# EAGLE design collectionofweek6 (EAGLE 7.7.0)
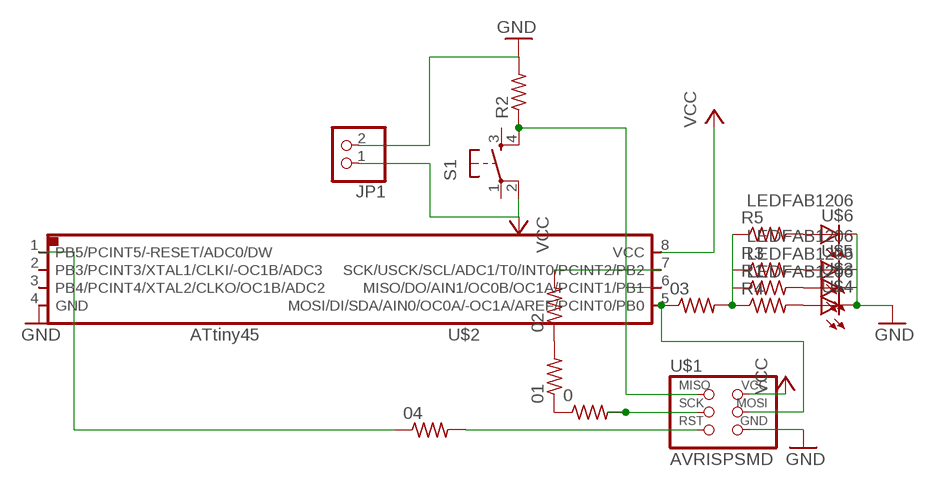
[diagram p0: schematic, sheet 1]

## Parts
0  RES-US1206FAB  [R1206FAB]
01  RES-US1206FAB  [R1206FAB]
02  RES-US1206FAB  [R1206FAB]
03  RES-US1206FAB  [R1206FAB]
04  RES-US1206FAB  [R1206FAB]
JP1  PINHD-1X2  [1X02]
R1  RES-US1206FAB  [R1206FAB]
R2  RES-US1206FAB  [R1206FAB]
R3  RES-US1206FAB  [R1206FAB]
R4  RES-US1206FAB  [R1206FAB]
R5  RES-US1206FAB  [R1206FAB]
S1  6MM_SWITCH6MM_SWITCH  [6MM_SWITCH]
U$1  AVRISPSMD  [2X03SMD]
U$2  ATTINY45SI  [SOIC8]
U$3  LEDFAB1206  [LED1206FAB]
U$4  LEDFAB1206  [LED1206FAB]
U$5  LEDFAB1206  [LED1206FAB]
U$6  LEDFAB1206  [LED1206FAB]

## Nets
GND: JP1.2 R2.2 U$1.6(GND) U$2.4(GND) U$3.2(C) U$4.2(C) U$5.2(C) U$6.2(C)
N$1: 03.1 U$1.4(MOSI) U$2.5(MOSI/DI/SDA/AIN0/OC0A/-OC1A/AREF/PCINT0/PB0)
N$2: R4.2 U$4.1(A)
N$3: R2.1 S1.4(S1) U$1.1(MISO) U$2.6(MISO/DO/AIN1/OC0B/OC1A/PCINT1/PB1)
N$4: 04.1 U$2.1(PB5/PCINT5/-RESET/ADC0/DW)
N$5: 03.2 R1.1 R3.1 R4.1 R5.1
N$6: 0.2 U$1.3(SCK)
N$7: R1.2 U$3.1(A)
N$8: R3.2 U$5.1(A)
N$9: R5.2 U$6.1(A)
N$10: 04.2 U$1.5(RST)
N$11: 0.1 01.1
N$12: 02.2 U$2.7(SCK/USCK/SCL/ADC1/T0/INT0/PCINT2/PB2)
N$13: 01.2 02.1
VCC: JP1.1 S1.2(P1) U$1.2(VCC) U$2.8(VCC)
Unconnected: S1.1(P) S1.3(S) U$2.2(PB3/PCINT3/XTAL1/CLKI/-OC1B/ADC3) U$2.3(PB4/PCINT4/XTAL2/CLKO/OC1B/ADC2)

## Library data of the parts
0 01-04 R1-R5 = fab:RES-US: Resistor (US Symbol)
JP1 = pinhead:PINHD-1X2: PIN HEADER
S1 = fab:6MM_SWITCH: OMRON SWITCH
U$1 = fab:AVRISP
U$2 = fab:ATTINY45
U$3-U$6 = fab:LED: LED

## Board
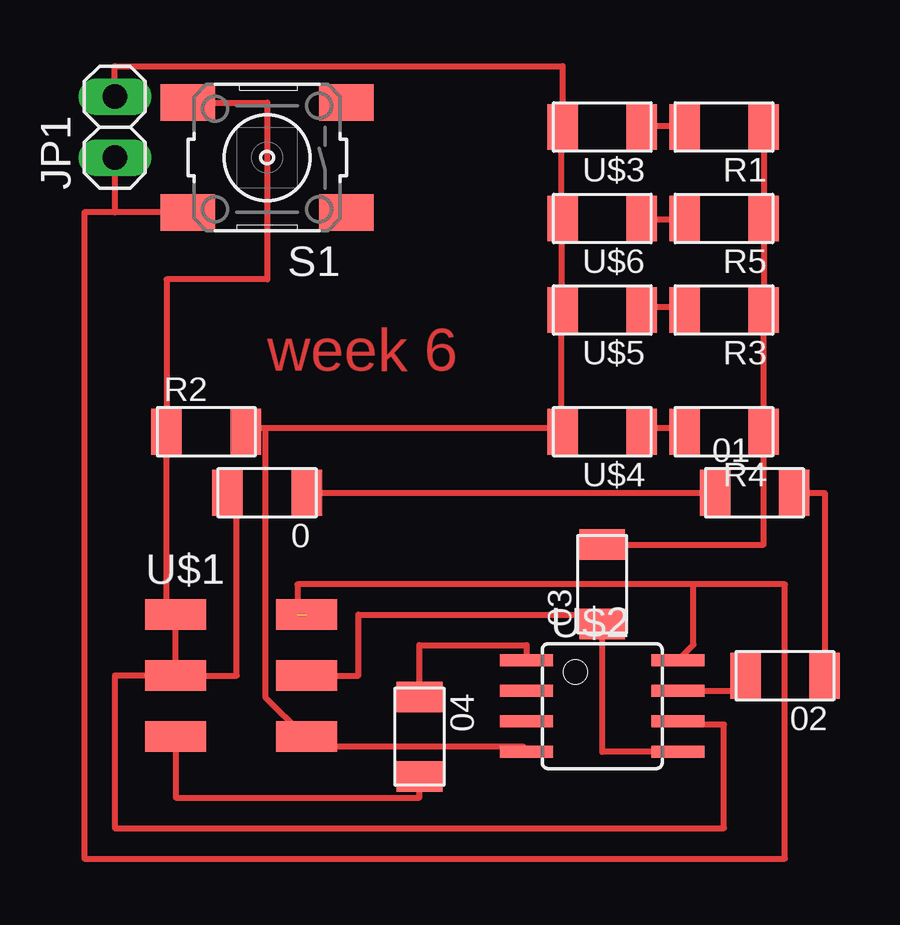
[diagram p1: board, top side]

No outline drawn. Coordinates in mm, seen from the top.
Copper layers (1*16): Top 0.035mm / dielectric 1.5mm / Bottom 0.035mm
Design rules "default": minimum track width 10mil, minimum drill 24mil, track to track 8mil, track to pad 8mil, pad to pad 8mil, via to via 8mil, smd to smd 8mil, copper to edge 40mil, drill to drill 8mil, minimum pad ring 10mil, minimum via ring 8mil, stop-mask expansion 4mil, vias tented up to drill 0mil, thermal gap 10mil

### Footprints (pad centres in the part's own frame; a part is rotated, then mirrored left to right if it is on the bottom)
R1206FAB = smd 1.27 x 1.905: 1 -1.651,0; 2 1.651,0
1X02 = drill 1.016 long: 1 -1.27,0; 2 1.27,0
6MM_SWITCH = smd 2.286 x 1.524: 1 -3.302,2.286; 2 3.302,2.286; 3 -3.302,-2.286; 4 3.302,-2.286
2X03SMD = smd 2.54 x 1.27: 1 -2.54,2.54; 2 2.92,2.54; 3 -2.54,0; 4 2.92,0; 5 -2.54,-2.54; 6 2.92,-2.54
SOIC8 = smd 0.5 x 2.2: 1 -1.905,-3.154; 2 -0.645,-3.154; 3 0.625,-3.154; 4 1.895,-3.154; 5 1.905,3.154; 6 0.635,3.154; 7 -0.635,3.154; 8 -1.905,3.154
LED1206FAB = smd 1.27 x 1.905: 1 -1.651,0; 2 1.651,0

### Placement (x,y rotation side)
0  7.62,16.51 180 top
01  27.94,16.51 0 top
02  29.21,8.89 180 top
03  21.59,12.7 90 top
04  13.97,6.35 270 top
JP1  1.27,31.75 90 top
R1  26.67,31.75 180 top
R2  5.08,19.05 0 top
R3  26.67,24.13 180 top
R4  26.67,19.05 180 top
R5  26.67,27.94 180 top
S1  7.62,30.48 180 top
U$1  6.35,8.89 0 top
U$2  21.59,7.62 270 top
U$3  21.59,31.75 180 top
U$4  21.59,19.05 180 top
U$5  21.59,24.13 180 top
U$6  21.59,27.94 180 top

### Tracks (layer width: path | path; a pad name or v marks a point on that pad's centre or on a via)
GND
  Top 0.254: U$2.4 18.29,5.94 9.6,5.94 9.37,6.17 U$1.6 9.14,6.4 7.54,8 7.54,19.2 | 19.89,19.2 7.54,19.2 | 7.54,19.2 6.86,19.2 R2.2 | 19.89,19.2 19.89,24 U$5.2 19.89,24.23 19.89,27.89 U$6.2 19.89,28.12 19.89,31.55 U$3.2 19.94,34.29 1.27,34.29 JP1.2 | 19.89,19.2 U$4.2
N$1
  Top 0.254: 9.37,8.91 U$1.4 11.43,8.89 11.43,11.43 21.59,11.43 03.1 21.59,5.71 U$2.5
N$2
  Top 0.254: U$4.1 23.32,19.2 24.92,19.2 R4.2
N$3
  Top 0.254: U$1.1 3.66,11.43 3.43,11.66 R2.1 3.43,25.4 7.62,25.4 7.62,32.77 S1.4 | U$2.6 24.92,6.86 26.67,6.86 26.67,2.54 1.27,2.54 1.27,8.89 3.81,8.89 U$1.1 | 3.89,11.43 U$1.1
N$4
  Top 0.254: 04.1 13.97,10.16 18.44,10.16 U$2.1
N$5
  Top 0.254: 03.2 28.32,14.35 R4.1 R3.1 R5.1 R1.1
N$6
  Top 0.254: 3.89,8.69 U$1.3 6.35,8.89 6.35,16.51 0.2
N$7
  Top 0.254: U$3.1 23.32,31.77 24.92,31.77 R1.2
N$8
  Top 0.254: U$5.1 23.32,24.23 24.92,24.23 R3.2
N$9
  Top 0.254: U$6.1 23.32,27.89 24.92,27.89 R5.2
N$10
  Top 0.254: U$1.5 3.81,3.81 13.97,3.81 04.2
N$11
  Top 0.254: 0.1 01.1
N$12
  Top 0.254: U$2.7 27.56,8.26 02.2
N$13
  Top 0.254: 01.2 30.86,16.51 02.1
VCC  (1 unrouted)
  Top 0.254: 25.4,12.7 29.21,12.7 29.21,1.27 0,1.27 0,28.19 1.27,28.19 | 25.4,12.7 8.89,12.7 8.89,11.43 | U$2.8 25.4,10.18 25.4,12.7 | S1.2 1.27,28.19 | JP1.1 1.27,28.19

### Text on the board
Top: week 6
